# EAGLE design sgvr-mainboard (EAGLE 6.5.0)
CNAME: SGVR Mainboard with Encoder; CREVISION: 1; DESIGNER: Rian Wardana

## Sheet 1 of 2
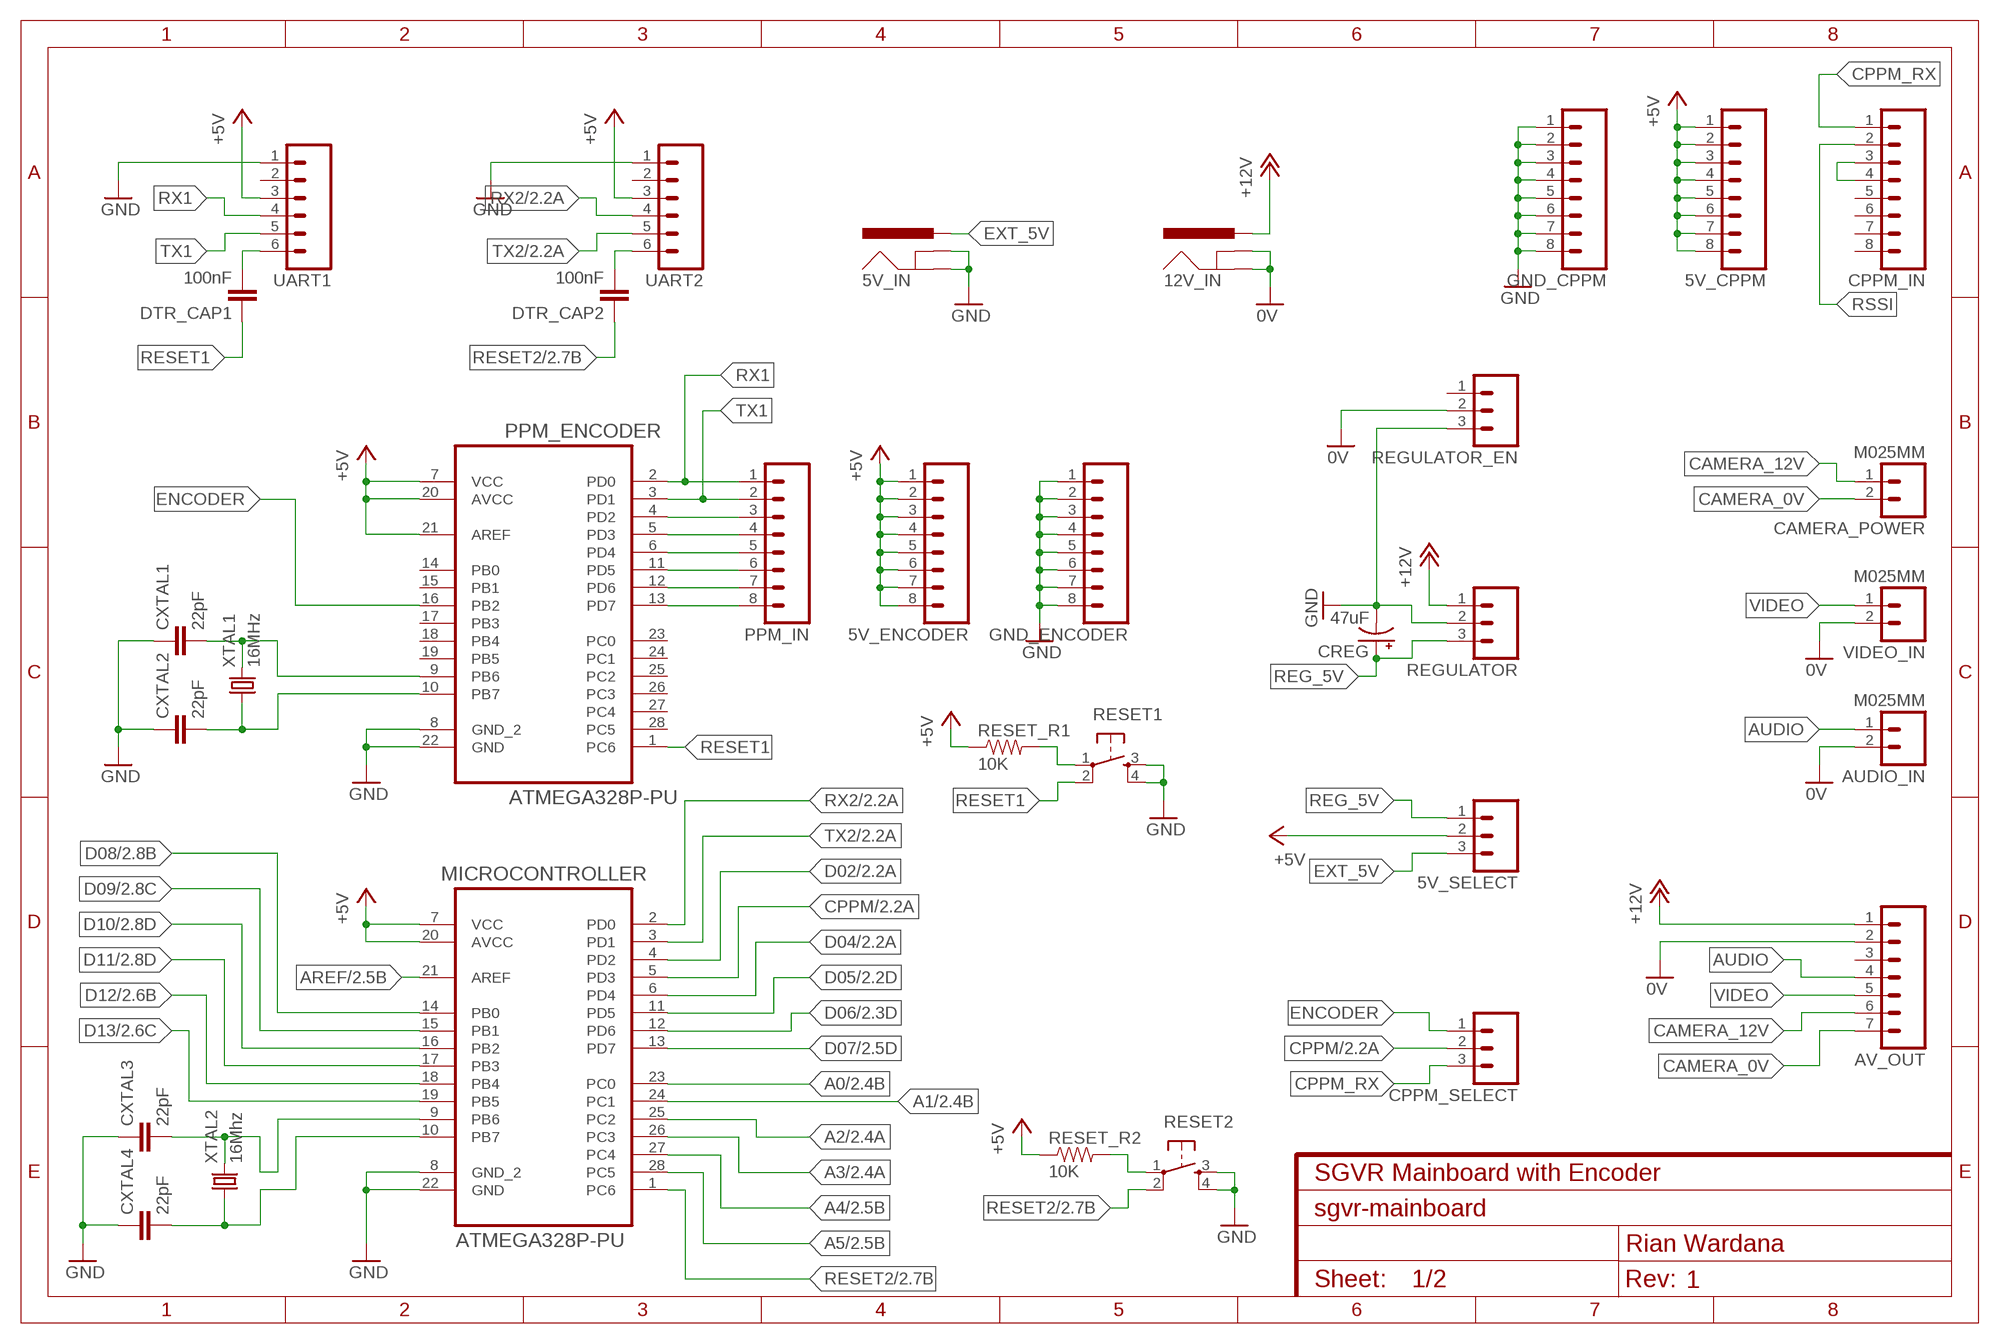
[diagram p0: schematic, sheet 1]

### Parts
5V_CPPM  M08LOCK  [1X08_LOCK]
5V_ENCODER  M08LOCK  [1X08_LOCK]
5V_IN  POWER_JACKPTH_LOCK  [POWER_JACK_PTH_LOCK]
5V_SELECT  M03LOCK_LONGPADS  [1X03_LOCK_LONGPADS]
12V_IN  POWER_JACKPTH_LOCK  [POWER_JACK_PTH_LOCK]
AUDIO_IN  M025MM  [SCREWTERMINAL-5MM-2]
AV_OUT  M07LOCK_LONGPADS  [1X07_LOCK_LONGPADS]
CAMERA_POWER  M025MM  [SCREWTERMINAL-5MM-2]
CPPM_IN  M08LOCK  [1X08_LOCK]
CPPM_SELECT  M03LOCK_LONGPADS  [1X03_LOCK_LONGPADS]
CREG  47uF  CAP_POLPTH1  [CPOL-RADIAL-100UF-25V]
CXTAL1  22pF  CAPPTH  [CAP-PTH-SMALL]
CXTAL2  22pF  CAPPTH  [CAP-PTH-SMALL]
CXTAL3  22pF  CAPPTH  [CAP-PTH-SMALL]
CXTAL4  22pF  CAPPTH  [CAP-PTH-SMALL]
DTR_CAP1  100nF  CAPPTH  [CAP-PTH-SMALL]
DTR_CAP2  100nF  CAPPTH  [CAP-PTH-SMALL]
GND_CPPM  M08LOCK  [1X08_LOCK]
GND_ENCODER  M08LOCK  [1X08_LOCK]
MICROCONTROLLER  ATMEGA328P-PU  [DIP254P762X457-28]
PPM_ENCODER  ATMEGA328P-PU  [DIP254P762X457-28]
PPM_IN  M08LOCK  [1X08_LOCK]
REGULATOR  M03LOCK_LONGPADS  [1X03_LOCK_LONGPADS]
REGULATOR_EN  M03LOCK_LONGPADS  [1X03_LOCK_LONGPADS]
RESET1  TAC_SWITCHPTH  [TACTILE-PTH]
RESET2  TAC_SWITCHPTH  [TACTILE-PTH]
RESET_R1  10K  RESISTORAXIAL-0.3  [AXIAL-0.3]
RESET_R2  10K  RESISTORAXIAL-0.3  [AXIAL-0.3]
UART1  M06LOCK_LONGPADS  [1X06_LOCK_LONGPADS]
UART2  M06LOCK_LONGPADS  [1X06_LOCK_LONGPADS]
VIDEO_IN  M025MM  [SCREWTERMINAL-5MM-2]
XTAL1  16MHz  CRYSTALHC49UV  [HC49U-V]
XTAL2  16Mhz  CRYSTALHC49UV  [HC49U-V]

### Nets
+5V: 5V_CPPM.1 5V_CPPM.2 5V_CPPM.3 5V_CPPM.4 5V_CPPM.5 5V_CPPM.6 5V_CPPM.7 5V_CPPM.8 5V_ENCODER.1 5V_ENCODER.2 5V_ENCODER.3 5V_ENCODER.4 5V_ENCODER.5 5V_ENCODER.6 5V_ENCODER.7 5V_ENCODER.8 5V_SELECT.2 MICROCONTROLLER.7(VCC) MICROCONTROLLER.20(AVCC) PPM_ENCODER.7(VCC) PPM_ENCODER.20(AVCC) PPM_ENCODER.21(AREF) RESET_R1.P$1 RESET_R2.P$1 UART1.3 UART2.3 ; also sheet 2
+12V: 12V_IN.PWR AV_OUT.1 REGULATOR.1
A0: MICROCONTROLLER.23(PC0) ; also sheet 2
A1: MICROCONTROLLER.24(PC1) ; also sheet 2
A2: MICROCONTROLLER.25(PC2) ; also sheet 2
A3: MICROCONTROLLER.26(PC3) ; also sheet 2
A4: MICROCONTROLLER.27(PC4) ; also sheet 2
A5: MICROCONTROLLER.28(PC5) ; also sheet 2
AREF: MICROCONTROLLER.21(AREF) ; also sheet 2
AUDIO: AUDIO_IN.1 AV_OUT.4
CAMERA_0V: AV_OUT.7 CAMERA_POWER.2
CAMERA_12V: AV_OUT.6 CAMERA_POWER.1
CPPM: CPPM_SELECT.2 MICROCONTROLLER.5(PD3) ; also sheet 2
CPPM_RX: CPPM_IN.1 CPPM_SELECT.3
D02: MICROCONTROLLER.4(PD2) ; also sheet 2
D04: MICROCONTROLLER.6(PD4) ; also sheet 2
D05: MICROCONTROLLER.11(PD5) ; also sheet 2
D06: MICROCONTROLLER.12(PD6) ; also sheet 2
D07: MICROCONTROLLER.13(PD7) ; also sheet 2
D08: MICROCONTROLLER.14(PB0) ; also sheet 2
D09: MICROCONTROLLER.15(PB1) ; also sheet 2
D10: MICROCONTROLLER.16(PB2) ; also sheet 2
D11: MICROCONTROLLER.17(PB3) ; also sheet 2
D12: MICROCONTROLLER.18(PB4) ; also sheet 2
D13: MICROCONTROLLER.19(PB5) ; also sheet 2
DTR: DTR_CAP1.2 UART1.6
DTR1: DTR_CAP2.2 UART2.6
ENCODER: CPPM_SELECT.1 PPM_ENCODER.16(PB2)
EXT_5V: 5V_IN.PWR 5V_SELECT.3
GND: 5V_IN.GND 5V_IN.GNDBREAK CREG.2(-) CXTAL1.1 CXTAL2.1 CXTAL3.1 CXTAL4.1 GND_CPPM.1 GND_CPPM.2 GND_CPPM.3 GND_CPPM.4 GND_CPPM.5 GND_CPPM.6 GND_CPPM.7 GND_CPPM.8 GND_ENCODER.1 GND_ENCODER.2 GND_ENCODER.3 GND_ENCODER.4 GND_ENCODER.5 GND_ENCODER.6 GND_ENCODER.7 GND_ENCODER.8 MICROCONTROLLER.8(GND_2) MICROCONTROLLER.22(GND) PPM_ENCODER.8(GND_2) PPM_ENCODER.22(GND) REGULATOR.2 REGULATOR_EN.3 RESET1.3 RESET1.4 RESET2.3 RESET2.4 UART1.1 UART2.1 ; also sheet 2
GROUND12: 12V_IN.GND 12V_IN.GNDBREAK AUDIO_IN.2 AV_OUT.2 REGULATOR_EN.2 VIDEO_IN.2 ; supply symbol labelled 0V
N$1: CXTAL1.2 PPM_ENCODER.9(PB6) XTAL1.2
N$2: CXTAL2.2 PPM_ENCODER.10(PB7) XTAL1.1
N$3: CXTAL3.2 MICROCONTROLLER.9(PB6) XTAL2.2
N$4: CXTAL4.2 MICROCONTROLLER.10(PB7) XTAL2.1
N$7: PPM_ENCODER.4(PD2) PPM_IN.3
N$8: PPM_ENCODER.5(PD3) PPM_IN.4
N$9: PPM_ENCODER.6(PD4) PPM_IN.5
N$10: PPM_ENCODER.11(PD5) PPM_IN.6
N$11: PPM_ENCODER.12(PD6) PPM_IN.7
N$12: PPM_ENCODER.13(PD7) PPM_IN.8
N$13: RESET2.1 RESET_R2.P$2
N$14: CPPM_IN.3 CPPM_IN.4
N$15: RESET1.1 RESET_R1.P$2
REG_5V: 5V_SELECT.1 CREG.1(+) REGULATOR.3
RESET1: DTR_CAP1.1 PPM_ENCODER.1(PC6) RESET1.2
RESET2: DTR_CAP2.1 MICROCONTROLLER.1(PC6) RESET2.2 ; also sheet 2
RSSI: CPPM_IN.2
RX1: PPM_ENCODER.2(PD0) PPM_IN.1 UART1.4
RX2: MICROCONTROLLER.2(PD0) UART2.4 ; also sheet 2
TX1: PPM_ENCODER.3(PD1) PPM_IN.2 UART1.5
TX2: MICROCONTROLLER.3(PD1) UART2.5 ; also sheet 2
VIDEO: AV_OUT.5 VIDEO_IN.1
Unconnected: AV_OUT.3 CPPM_IN.5 CPPM_IN.6 CPPM_IN.7 CPPM_IN.8 PPM_ENCODER.14(PB0) PPM_ENCODER.15(PB1) PPM_ENCODER.17(PB3) PPM_ENCODER.18(PB4) PPM_ENCODER.19(PB5) PPM_ENCODER.23(PC0) PPM_ENCODER.24(PC1) PPM_ENCODER.25(PC2) PPM_ENCODER.26(PC3) PPM_ENCODER.27(PC4) PPM_ENCODER.28(PC5) REGULATOR_EN.1 UART1.2 UART2.2

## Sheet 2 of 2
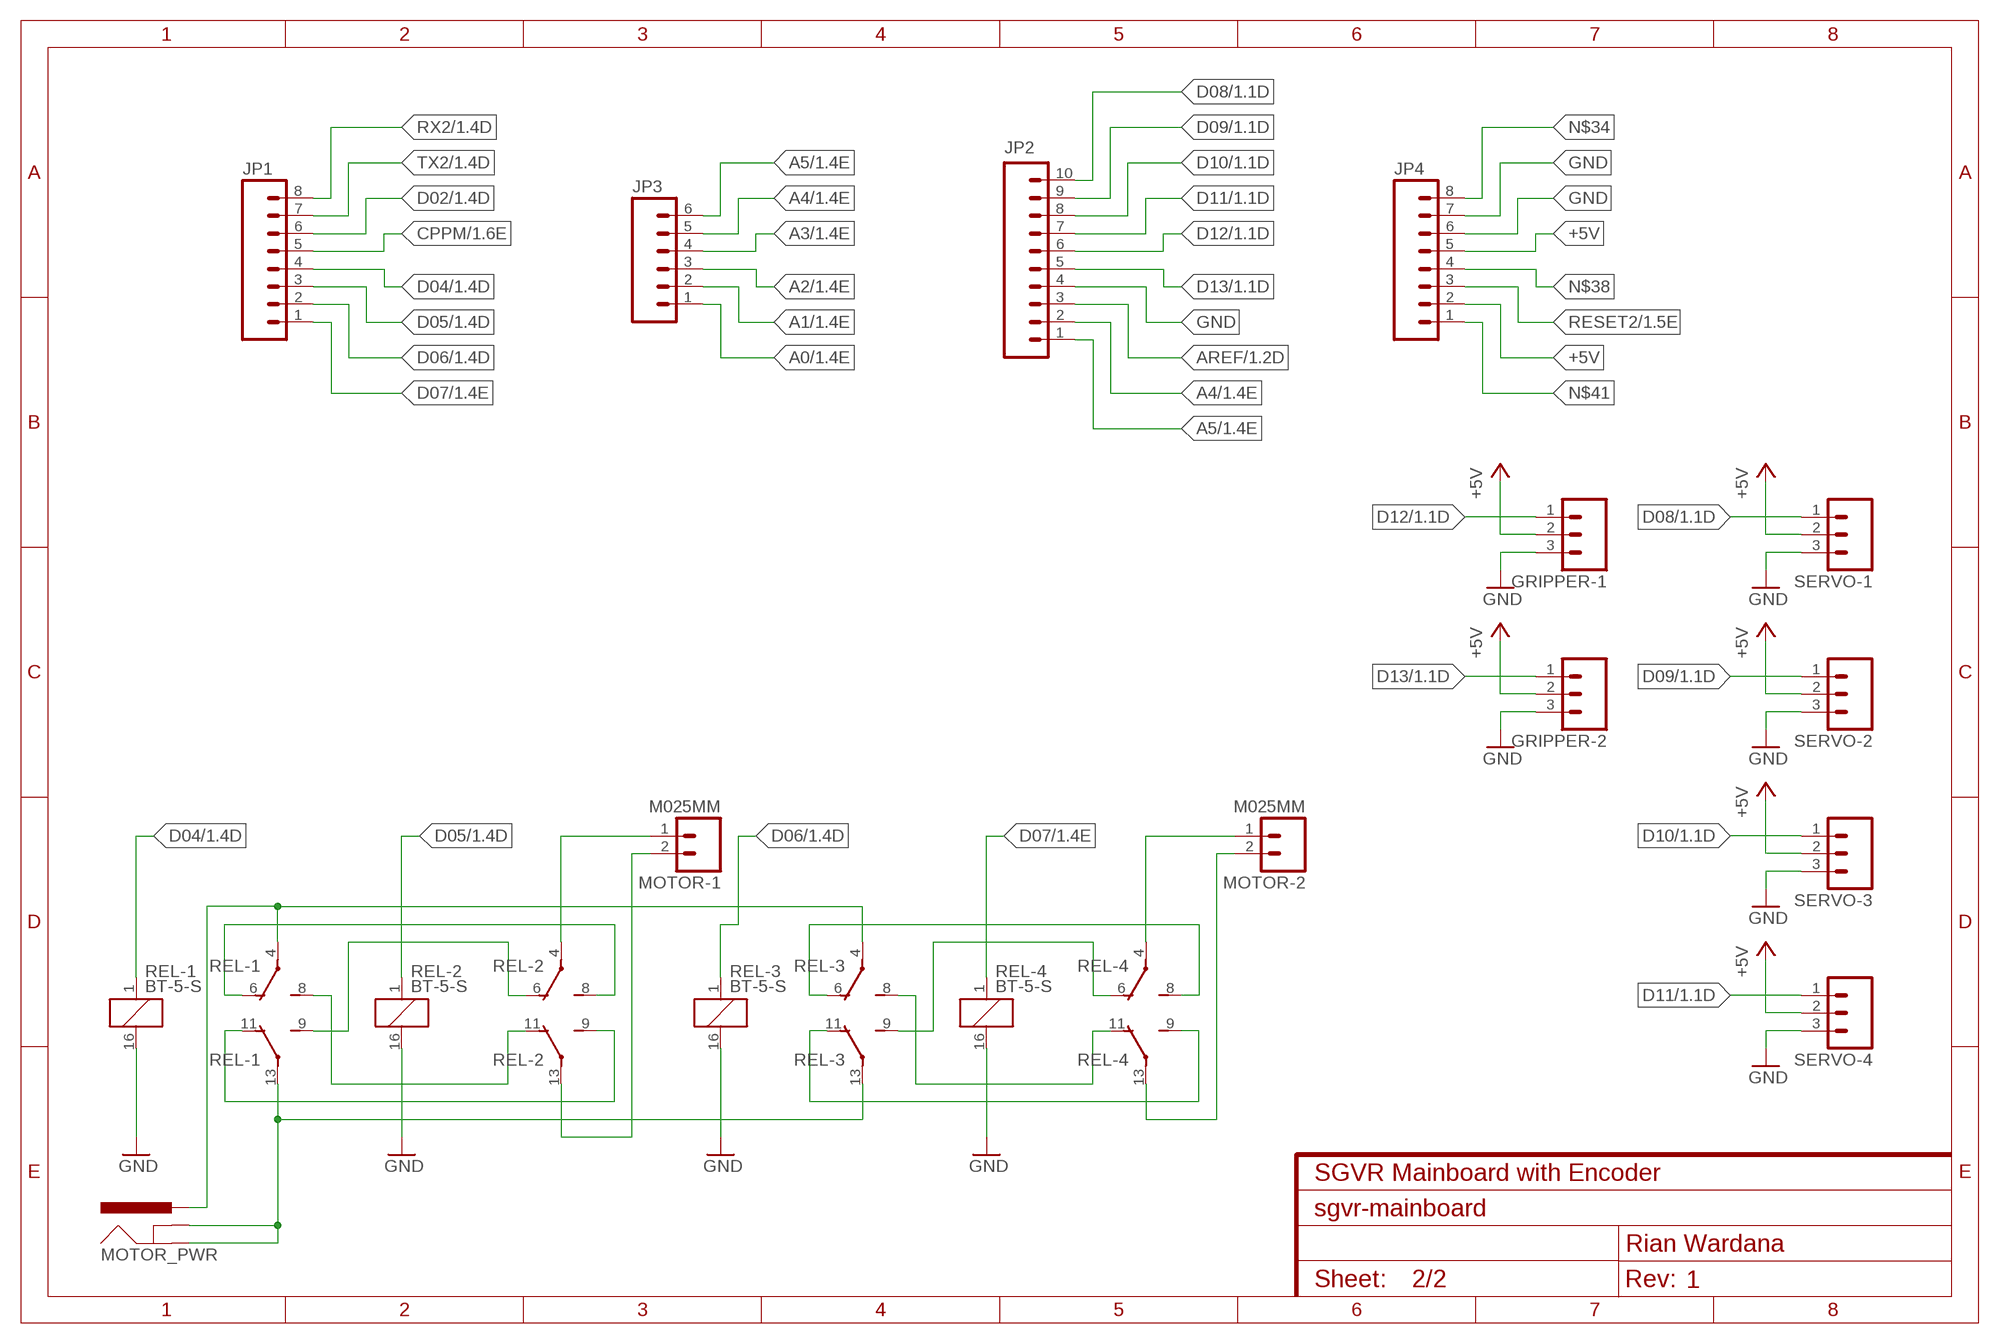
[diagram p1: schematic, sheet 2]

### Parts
GRIPPER-1  M03LOCK_LONGPADS  [1X03_LOCK_LONGPADS]
GRIPPER-2  M03LOCK_LONGPADS  [1X03_LOCK_LONGPADS]
JP1  M08LOCK_LONGPADS  [1X08_LOCK_LONGPADS]
JP2  M10LOCK_LONGPADS  [1X10_LOCK_LONGPADS]
JP3  M06LOCK_LONGPADS  [1X06_LOCK_LONGPADS]
JP4  M08LOCK_LONGPADS  [1X08_LOCK_LONGPADS]
MOTOR-1  M025MM  [SCREWTERMINAL-5MM-2]
MOTOR-2  M025MM  [SCREWTERMINAL-5MM-2]
MOTOR_PWR  POWER_JACKPTH_LOCK  [POWER_JACK_PTH_LOCK]
REL-1  BT-5-S  [BT-XX-S]
REL-2  BT-5-S  [BT-XX-S]
REL-3  BT-5-S  [BT-XX-S]
REL-4  BT-5-S  [BT-XX-S]
SERVO-1  M03LOCK_LONGPADS  [1X03_LOCK_LONGPADS]
SERVO-2  M03LOCK_LONGPADS  [1X03_LOCK_LONGPADS]
SERVO-3  M03LOCK_LONGPADS  [1X03_LOCK_LONGPADS]
SERVO-4  M03LOCK_LONGPADS  [1X03_LOCK_LONGPADS]

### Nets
+5V: GRIPPER-1.2 GRIPPER-2.2 JP4.2 JP4.5 SERVO-1.2 SERVO-2.2 SERVO-3.2 SERVO-4.2 ; also sheet 1
A0: JP3.1 ; also sheet 1
A1: JP3.2 ; also sheet 1
A2: JP3.3 ; also sheet 1
A3: JP3.4 ; also sheet 1
A4: JP2.2 JP3.5 ; also sheet 1
A5: JP2.1 JP3.6 ; also sheet 1
AREF: JP2.3 ; also sheet 1
CPPM: JP1.5 ; also sheet 1
D02: JP1.6 ; also sheet 1
D04: JP1.4 REL-1.1 ; also sheet 1
D05: JP1.3 REL-2.1 ; also sheet 1
D06: JP1.2 REL-3.1 ; also sheet 1
D07: JP1.1 REL-4.1 ; also sheet 1
D08: JP2.10 SERVO-1.1 ; also sheet 1
D09: JP2.9 SERVO-2.1 ; also sheet 1
D10: JP2.8 SERVO-3.1 ; also sheet 1
D11: JP2.7 SERVO-4.1 ; also sheet 1
D12: GRIPPER-1.1 JP2.6 ; also sheet 1
D13: GRIPPER-2.1 JP2.5 ; also sheet 1
GND: GRIPPER-1.3 GRIPPER-2.3 JP2.4 JP4.6 JP4.7 REL-1.16 REL-2.16 REL-3.16 REL-4.16 SERVO-1.3 SERVO-2.3 SERVO-3.3 SERVO-4.3 ; also sheet 1
N$5: REL-3.11(-2:O) REL-4.9(-2:S)
N$6: REL-3.6(-1:O) REL-4.8(-1:S)
N$18: MOTOR-2.1 REL-4.4(-1:P)
N$19: MOTOR-2.2 REL-4.13(-2:P)
N$20: REL-3.9(-2:S) REL-4.6(-1:O)
N$21: REL-3.8(-1:S) REL-4.11(-2:O)
N$22: REL-1.11(-2:O) REL-2.9(-2:S)
N$23: REL-1.6(-1:O) REL-2.8(-1:S)
N$24: MOTOR_PWR.PWR REL-1.4(-1:P) REL-3.4(-1:P)
N$25: MOTOR_PWR.GND MOTOR_PWR.GNDBREAK REL-1.13(-2:P) REL-3.13(-2:P)
N$26: MOTOR-1.1 REL-2.4(-1:P)
N$27: MOTOR-1.2 REL-2.13(-2:P)
N$28: REL-1.9(-2:S) REL-2.6(-1:O)
N$29: REL-1.8(-1:S) REL-2.11(-2:O)
N$34: JP4.8
N$38: JP4.4
N$41: JP4.1
RESET2: JP4.3 ; also sheet 1
RX2: JP1.8 ; also sheet 1
TX2: JP1.7 ; also sheet 1

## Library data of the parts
5V_CPPM 5V_ENCODER CPPM_IN GND_CPPM GND_ENCODER JP1 JP4 PPM_IN = SparkFun-Connectors:M08: Header 8 Standard 8-pin 0.1" header. Use with straight break away headers (SKU : PRT-00116), right angle break away headers (PRT-00553), swiss pins (PRT-00743), machine pins (PRT-00117), and female headers (PRT-00115).
5V_IN 12V_IN MOTOR_PWR = SparkFun-Connectors:POWER_JACK: Power Jack This is the standard 5.5mm barrel jack for power. The PTH is the most common, proven, reliable, footprint. The Slot footprint only works if the mill layer is transmitted to the PCB fab house so be warned. Mating wall wart : TOL-00298 (and others); PROD_ID: PRT-00119
5V_SELECT CPPM_SELECT GRIPPER-1 GRIPPER-2 REGULATOR REGULATOR_EN SERVO-1-SERVO-4 = SparkFun-Connectors:M03: Header 3 Standard 3-pin 0.1" header. Use with straight break away headers (SKU : PRT-00116), right angle break away headers (PRT-00553), swiss pins (PRT-00743), machine pins (PRT-00117), and female headers (PRT-00115). Molex polarized connector foot print use with SKU : PRT-08232 with associated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
AUDIO_IN CAMERA_POWER MOTOR-1 MOTOR-2 VIDEO_IN = SparkFun-Connectors:M02: Standard 2-pin 0.1" header. Use with
AV_OUT = SparkFun-Connectors:M07: Header 7 Standard 7-pin 0.1" header. Use with straight break away headers (SKU : PRT-00116), right angle break away headers (PRT-00553), swiss pins (PRT-00743), machine pins (PRT-00117), and female headers (PRT-00115). NOTES ON THE VARIANTS LOCK and LOCK_LONGPADS... This footprint was designed to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
CREG = SparkFun-Passives:CAP_POL: Capacitor Polarized
CXTAL1 CXTAL2 = SparkFun-Passives:CAP: Capacitor
CXTAL3 CXTAL4 DTR_CAP1 DTR_CAP2 = SparkFun-Capacitors:CAP: Capacitor
JP2 = SparkFun-Connectors:M10: Header 10 Standard 10-pin 0.1" header. Use with straight break away headers (SKU : PRT-00116), right angle break away headers (PRT-00553), swiss pins (PRT-00743), machine pins (PRT-00117), and female headers (PRT-00115).
JP3 UART1 UART2 = SparkFun-Connectors:M06: Header 6 Standard 6-pin 0.1" header. Use with straight break away headers (SKU : PRT-00116), right angle break away headers (PRT-00553), swiss pins (PRT-00743), machine pins (PRT-00117), and female headers (PRT-00115). Molex polarized connector foot print use with SKU : PRT-08094 with associated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
MICROCONTROLLER PPM_ENCODER = Atmel_By_element14_Batch_1-00:ATMEGA328P-PU: 8-bit Microcontroller with In-System Programmable Flash; MPN: ATMEGA328P-PU; OC_FARNELL: 1715487; OC_NEWARK: 15R0268; PACKAGE: PDIP-28; SUPPLIER: Atmel
REL-1-REL-4 = relay:BT-*-S: KLEIN RELAIS WASCHDICHT 2 Wechsler Distriibutor: Conrad Electronic, Bestell Nr.: 505226-13 - 24V 505226-13 - 5V 505170-13 - 12V 505170-13 - 48V Bestar Electric Ltd. Source: http://www2.produktinfo.conrad.com/datenblaetter/500000-524999/505226-da-01-en-Kleinrelais_waschdicht_24V.pdf; OC_FARNELL: unknown; OC_NEWARK: unknown
RESET1 RESET2 = SparkFun-Electromechanical:TAC_SWITCH: Momentary Switch Button commonly used for reset or general input. Spark Fun Electronics SKU : COM-00097 SMT- SWCH-08247
RESET_R1 RESET_R2 = SparkFun-Resistors:RESISTOR: Resistor
XTAL1 XTAL2 = SparkFun-FreqCtrl:CRYSTAL: Various standard crystals. Proven footprints. Spark Fun Electronics SKU : COM-00534

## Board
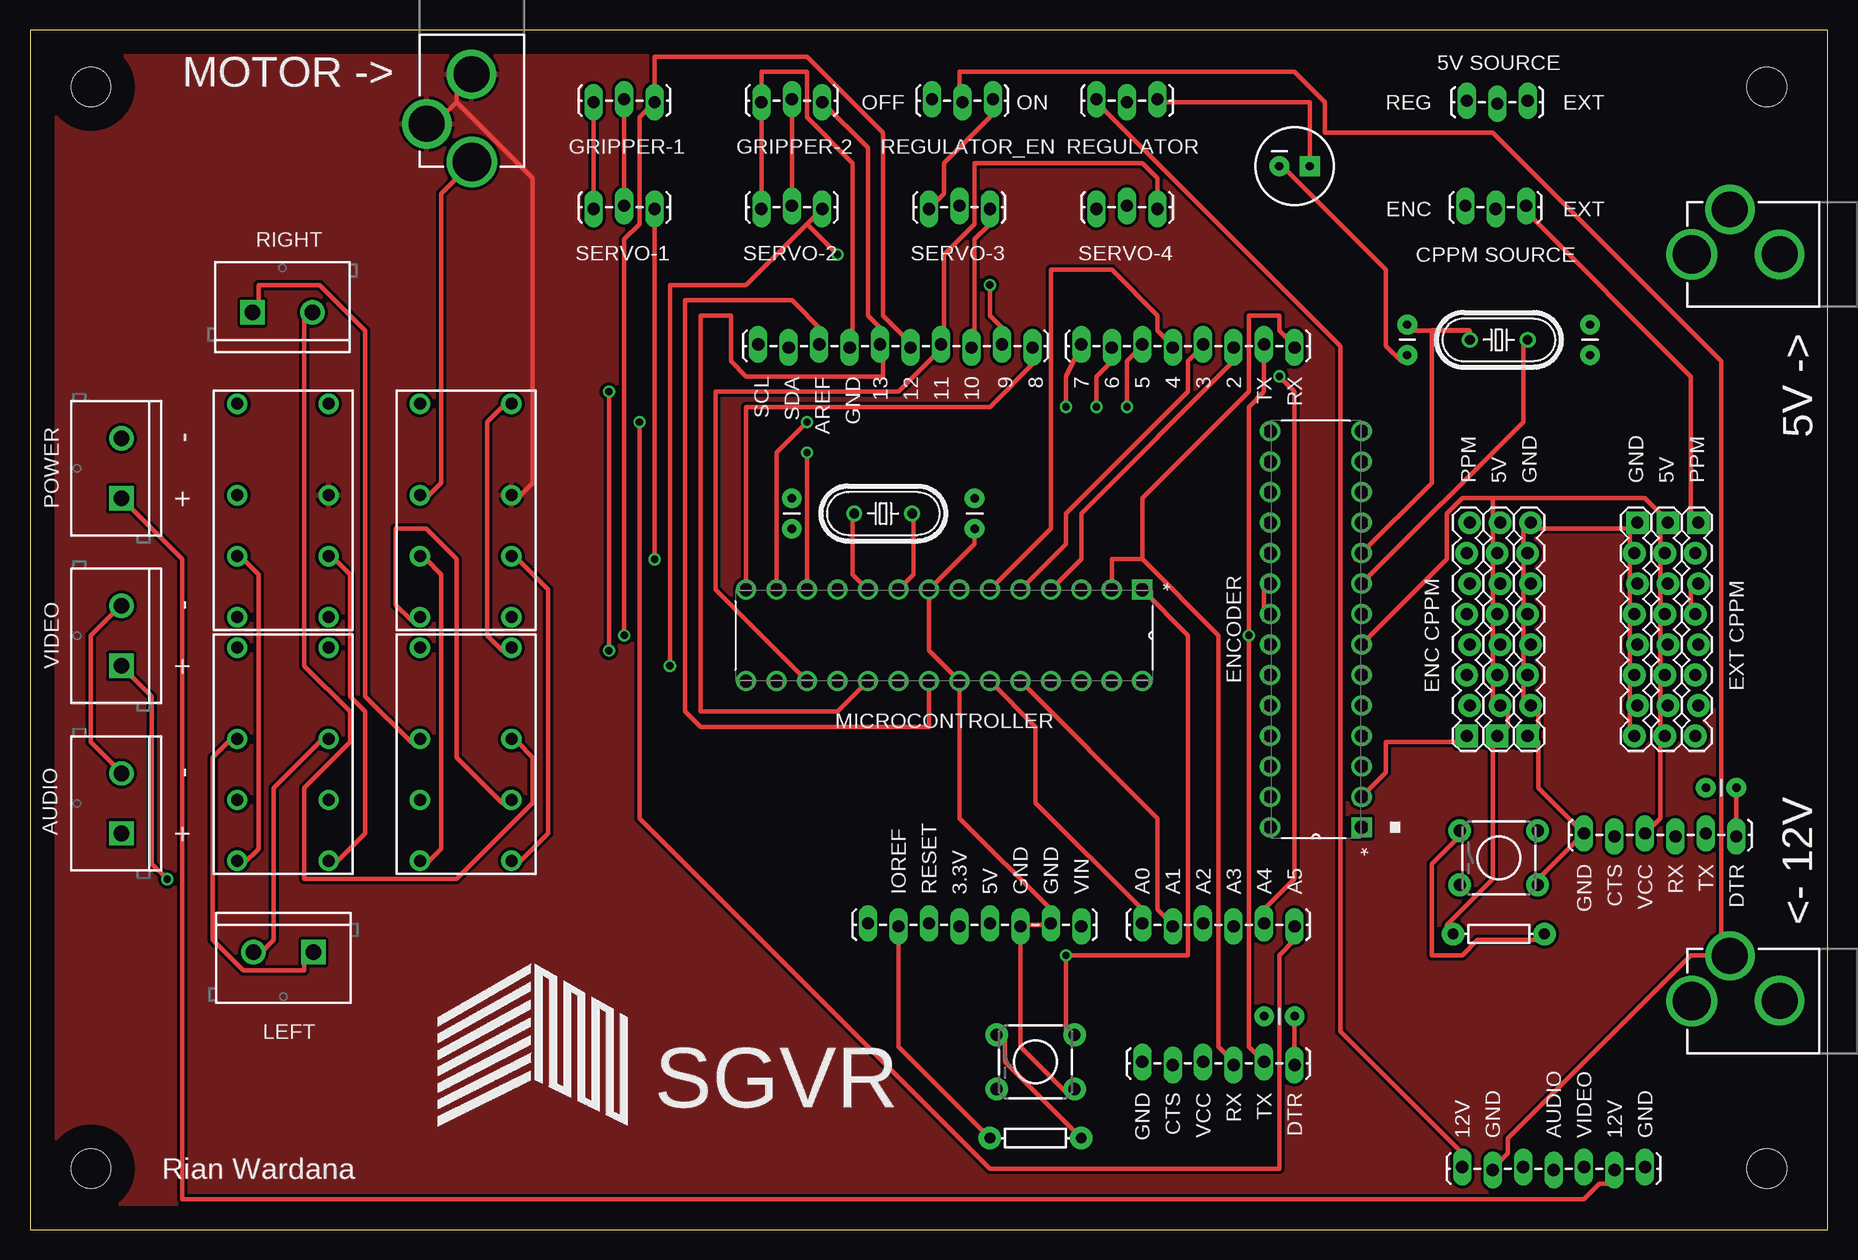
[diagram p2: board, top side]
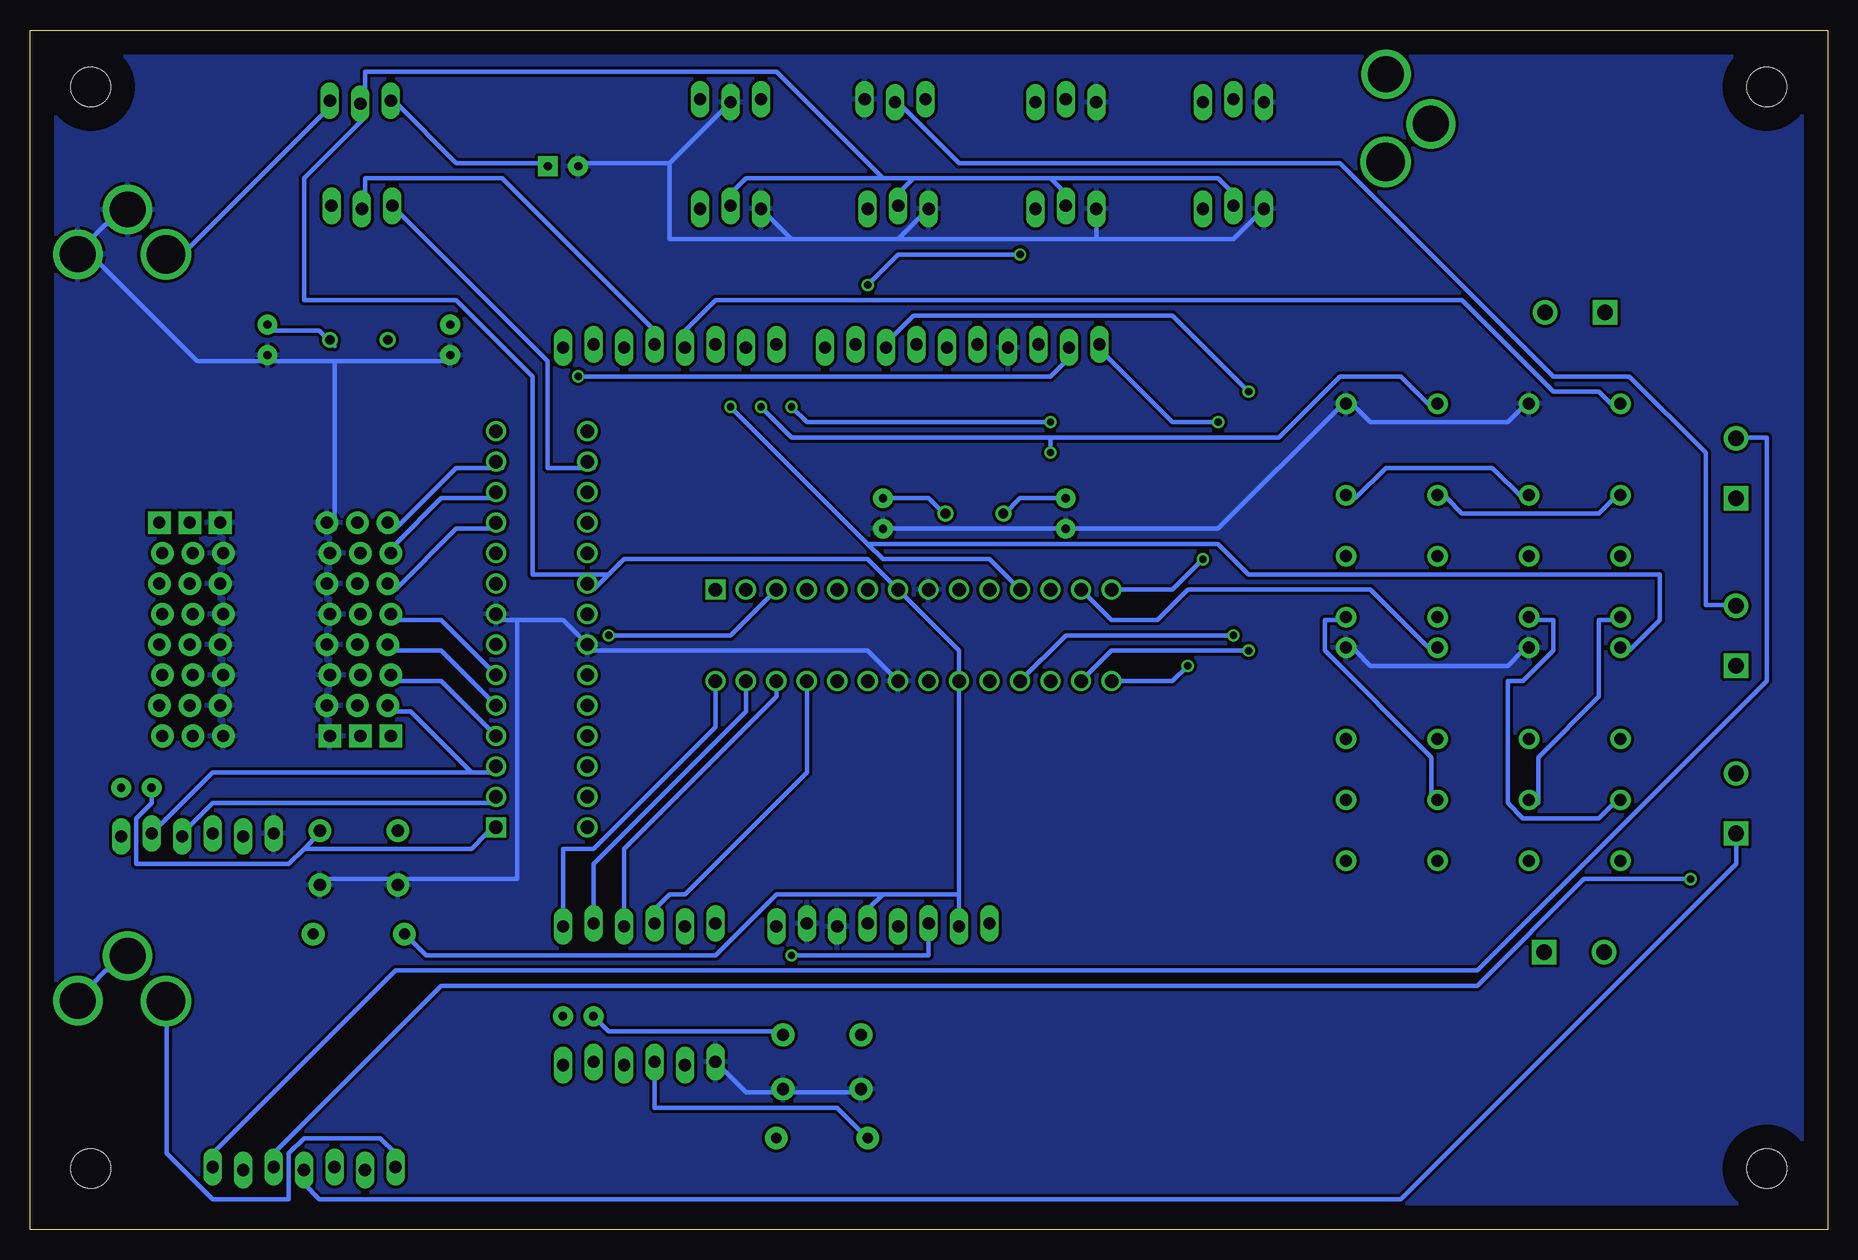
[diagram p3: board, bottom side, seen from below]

Size 149.84 x 100 mm. Coordinates in mm from the lower left corner, seen from the top.
Outline: 0,0 149.84,0 149.84,100 0,100 0,0
Copper layers (1*16): Top 0.035mm / dielectric 1.5mm / Bottom 0.035mm
Design rules "Mazmood *": minimum track width 15mil, minimum drill 24mil, track to track 10mil, track to pad 10mil, pad to pad 10mil, via to via 10mil, smd to smd 10mil, copper to edge 2mm, drill to drill 10mil, minimum pad ring 10mil, minimum via ring 8mil, stop-mask expansion 4mil, vias tented up to drill 0mil, thermal gap 10mil

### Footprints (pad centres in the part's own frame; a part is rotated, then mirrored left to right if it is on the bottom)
1X08_LOCK = drill 1.016 pad 1.88 square: 1 0,0.127 | drill 1.016 pad 1.88: 2 2.54,-0.127; 3 5.08,0.127; 4 7.62,-0.127; 5 10.16,0.127; 6 12.7,-0.127; 7 15.24,0.127; 8 17.78,-0.127
POWER_JACK_PTH_LOCK = drill 2.997 pad 4.115: GND 0.025,6.557; GNDBREAK 3.762,10.7 | drill 3.2 pad 4.115: PWR 0,13.878
1X03_LOCK_LONGPADS = drill 1.016 long: 1 0,0; 2 2.54,-0.254; 3 5.08,0
SCREWTERMINAL-5MM-2 = drill 1.3 pad 2.032 square: 1 0,0 | drill 1.3 pad 2.032: 2 5,0
1X07_LOCK_LONGPADS = drill 1.016 long: 1 0,0.127; 2 2.54,-0.127; 3 5.08,0.127; 4 7.62,-0.127; 5 10.16,0.127; 6 12.7,-0.127; 7 15.24,0.127
CPOL-RADIAL-100UF-25V = drill 0.7 pad 1.651 square: 1 1.27,0 | drill 0.7 pad 1.651: 2 -1.27,0
CAP-PTH-SMALL = drill 0.7 pad 1.651: 1 0,0; 2 2.54,0
1X08_LOCK_LONGPADS = drill 1.016 long: 1 0,0.127; 2 2.54,-0.127; 3 5.08,0.127; 4 7.62,-0.127; 5 10.16,0.127; 6 12.7,-0.127; 7 15.24,0.127; 8 17.78,-0.127
1X10_LOCK_LONGPADS = drill 1.016 long: 1 0,0.127; 2 2.54,-0.127; 3 5.08,0.127; 4 7.62,-0.127; 5 10.16,0.127; 6 12.7,-0.127; 7 15.24,0.127; 8 17.78,-0.127; 9 20.32,0.127; 10 22.86,-0.127
1X06_LOCK_LONGPADS = drill 1.016 long: 1 0,0; 2 2.54,-0.254; 3 5.08,0; 4 7.62,-0.254; 5 10.16,0; 6 12.7,-0.254
DIP254P762X457-28 = drill 1.118 square: 1 -7.62,33.02 | drill 1.118: 2 -7.62,30.48; 3 -7.62,27.94; 4 -7.62,25.4; 5 -7.62,22.86; 6 -7.62,20.32; 7 -7.62,17.78; 8 -7.62,15.24; 9 -7.62,12.7; 10 -7.62,10.16; 11 -7.62,7.62; 12 -7.62,5.08; 13 -7.62,2.54; 14 -7.62,0; 15 0,0; 16 0,2.54; 17 0,5.08; 18 0,7.62; 19 0,10.16; 20 0,12.7; 21 0,15.24; 22 0,17.78; 23 0,20.32; 24 0,22.86; 25 0,25.4; 26 0,27.94; 27 0,30.48; 28 0,33.02
BT-XX-S = drill 1 pad 1.7: 1 -8.89,-3.81; 4 -1.27,-3.81; 6 3.81,-3.81; 8 8.89,-3.81; 9 8.89,3.81; 11 3.81,3.81; 13 -1.27,3.81; 16 -8.89,3.81
TACTILE-PTH = drill 1.016 pad 1.88: 1 -3.251,2.261; 2 3.251,2.261; 3 -3.251,-2.261; 4 3.251,-2.261
AXIAL-0.3 = drill 0.9 pad 1.88: P$1 -3.81,0; P$2 3.81,0
STAND-OFF = hole 3.302: 0,0
HC49U-V = drill 0.813: 1 -2.413,0; 2 2.413,0

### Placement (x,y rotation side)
5V_CPPM  136.4,58.93 270 top
5V_ENCODER  122.43,41.15 90 top
5V_IN  152.4,81.28 90 top
5V_SELECT  119.76,94.11 0 top
12V_IN  152.4,19.05 90 top
AUDIO_IN  7.62,33.02 90 top
AV_OUT  119.38,5.08 0 top
CAMERA_POWER  7.62,60.96 90 top
CPPM_IN  138.94,58.93 270 top
CPPM_SELECT  119.63,85.34 0 top
CREG  105.41,88.65 0 top
CXTAL1  130.05,72.9 90 top
CXTAL2  114.81,72.9 90 top
CXTAL3  78.74,58.42 90 top
CXTAL4  63.5,58.42 90 top
DTR_CAP1  139.7,36.83 0 top
DTR_CAP2  102.87,17.78 0 top
GND_CPPM  133.86,58.93 270 top
GND_ENCODER  124.97,41.15 90 top
GRIPPER-1  52.07,93.98 180 top
GRIPPER-2  66.04,93.98 180 top
JP1  87.63,73.66 0 top
JP2  60.71,73.66 0 top
JP3  92.71,25.53 0 top
JP4  69.85,25.4 0 top
MICROCONTROLLER  59.69,45.72 270 top
MOTOR-1  23.62,23.11 180 top
MOTOR-2  18.54,76.45 0 top
MOTOR_PWR  36.83,102.87 180 top
PPM_ENCODER  103.38,66.55 180 top
PPM_IN  119.89,41.15 90 top
REGULATOR  88.9,94.23 0 top
REGULATOR_EN  75.18,94.23 0 top
REL-1  21.08,59.94 270 top
REL-2  21.08,39.62 270 top
REL-3  36.32,59.94 270 top
REL-4  36.32,39.62 270 top
RESET1  122.43,30.99 0 top
RESET2  83.82,13.97 0 top
RESET_R1  122.43,24.64 0 top
RESET_R2  83.82,7.62 0 top
SERVO-1  52.07,85.09 180 top
SERVO-2  66.04,85.09 180 top
SERVO-3  80.01,85.09 180 top
SERVO-4  93.98,85.09 180 top
U$1  [STAND-OFF]  5.08,5.08 0 top
U$2  [STAND-OFF]  5.08,95.25 0 top
U$3  [STAND-OFF]  144.78,5.08 0 top
U$4  [STAND-OFF]  144.78,95.25 0 top
UART1  129.54,33.02 0 top
UART2  92.71,13.97 0 top
VIDEO_IN  7.62,46.99 90 top
XTAL1  122.43,74.17 0 top
XTAL2  71.12,59.69 0 top

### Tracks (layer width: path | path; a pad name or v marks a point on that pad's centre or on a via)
+5V
  Top 0.381: GRIPPER-1.2 SERVO-1.2 | GRIPPER-2.2 SERVO-2.2 | 135.89,53.34 135.89,52.07 5V_CPPM.4 135.89,50.8 135.89,48.26 | 135.89,48.26 135.89,46.99 5V_CPPM.6 135.89,45.72 135.89,43.18 | UART1.3 135.89,34.29 135.89,40.64 5V_CPPM.8 135.89,41.91 135.89,43.18 | 135.89,43.18 5V_CPPM.7 | 135.89,48.26 5V_CPPM.5 | 135.89,53.34 135.89,55.88 5V_CPPM.2 135.89,57.15 135.89,58.42 5V_CPPM.1 135.89,59.69 134.62,60.96 121.92,60.96 | 135.89,53.34 5V_CPPM.3 | 121.92,60.96 119.38,60.96 118.11,59.69 118.11,55.88 PPM_ENCODER.7 110.49,48.26 | 121.92,58.42 121.92,60.96 | 121.92,58.42 121.92,57.15 5V_ENCODER.7 121.92,55.88 121.92,53.34 | 121.92,58.42 5V_ENCODER.8 | 121.92,53.34 121.92,52.07 5V_ENCODER.5 121.92,50.8 121.92,48.26 | 121.92,48.26 121.92,46.99 5V_ENCODER.3 121.92,45.72 121.92,43.18 5V_ENCODER.2 123.19,43.18 123.19,41.91 5V_ENCODER.1 121.92,40.64 121.92,29.21 118.11,25.4 RESET_R1.P$1 | 121.92,48.26 5V_ENCODER.4 | 121.92,53.34 5V_ENCODER.6 | PPM_ENCODER.21 102.87,50.8 102.87,53.34 PPM_ENCODER.20 | RESET_R2.P$1 72.39,15.24 JP4.2
  Bottom 0.381: 76.2,87.63 77.47,86.36 SERVO-3.2 | 64.77,87.63 76.2,87.63 | 64.77,87.63 63.5,86.36 SERVO-2.2 | 76.2,87.63 78.74,87.63 | 78.74,87.63 90.17,87.63 91.44,86.36 SERVO-4.2 | 78.74,87.63 87.63,96.52 121.92,96.52 121.92,93.98 5V_SELECT.2 121.92,92.71 127,87.63 127,77.47 114.3,77.47 107.95,71.12 107.95,54.61 101.6,54.61 | 64.77,87.63 50.8,87.63 49.53,86.36 SERVO-1.2 | UART2.3 97.79,10.16 82.55,10.16 RESET_R2.P$1 | 72.39,27.94 MICROCONTROLLER.20 72.39,48.26 MICROCONTROLLER.7 80.01,55.88 100.33,55.88 101.6,54.61 | 72.39,27.94 JP4.2 | 78.74,27.94 80.01,26.67 JP4.5 | 72.39,27.94 78.74,27.94 | 101.6,54.61 102.87,53.34 PPM_ENCODER.20 | RESET_R1.P$1 116.84,22.86 92.71,22.86 87.63,27.94 78.74,27.94
+12V
  Top 0.381: REGULATOR.1 88.9,93.98 109.22,73.66 109.22,16.51 119.38,6.35 AV_OUT.1
  Bottom 0.381: AV_OUT.1 119.38,6.35 120.65,7.62 127,7.62 128.27,6.35 128.27,2.54 134.62,2.54 138.43,6.35 138.43,19.05 12V_IN.PWR
A0
  Top 0.381: MICROCONTROLLER.23 83.82,41.91 83.82,35.56 92.71,26.67 JP3.1
A1
  Top 0.381: MICROCONTROLLER.24 93.98,34.29 93.98,26.67 95.25,25.4 JP3.2
A2
  Bottom 0.381: MICROCONTROLLER.25 85.09,38.1 95.25,27.94 96.52,27.94 97.79,26.67 JP3.3
A3
  Bottom 0.381: JP3.4 100.33,31.75 87.63,44.45 MICROCONTROLLER.26
A4  (via drill 0.61)
  Top 0.381: v104.14,71.12 105.41,69.85 105.41,29.21 102.87,26.67 JP3.5
  Bottom 0.381: JP3.5 102.87,30.48 90.17,43.18 MICROCONTROLLER.27 | v104.14,71.12 64.77,71.12 63.5,72.39 JP2.2
A5  (via drill 0.61)
  Top 0.381: v50.8,67.31 50.8,34.29 80.01,5.08 104.14,5.08 104.14,22.86 105.41,24.13 JP3.6
  Bottom 0.381: JP3.6 105.41,31.75 102.87,31.75 92.71,41.91 MICROCONTROLLER.28 | v50.8,67.31 54.61,67.31 60.96,73.66 JP2.1
AREF
  Top 0.381: MICROCONTROLLER.21 74.93,41.91 55.88,41.91 54.61,43.18 54.61,77.47 63.5,77.47 66.04,74.93 JP2.3
AUDIO
  Bottom 0.381: AUDIO_IN.1 7.62,30.48 35.56,2.54 125.73,2.54 127,3.81 AV_OUT.4
CAMERA_0V
  Bottom 0.381: AV_OUT.7 134.62,6.35 119.38,21.59 29.21,21.59 5.08,45.72 5.08,66.04 7.62,66.04 CAMERA_POWER.2
CAMERA_12V
  Top 0.381: CAMERA_POWER.1 12.7,55.88 12.7,2.54 129.54,2.54 130.81,3.81 132.08,3.81 AV_OUT.6
CPPM
  Top 0.381: MICROCONTROLLER.5 86.36,57.15 86.36,59.69 96.52,69.85 96.52,72.39 97.79,73.66 JP1.5
  Bottom 0.381: CPPM_SELECT.2 121.92,85.09 121.92,87.63 110.49,87.63 97.79,74.93 JP1.5
CPPM_RX
  Top 0.381: CPPM_SELECT.3 124.46,85.09 138.43,71.12 138.43,59.69 CPPM_IN.1
D02
  Top 0.381: MICROCONTROLLER.4 87.63,55.88 87.63,59.69 100.33,72.39 JP1.6
D04
  Top 0.381: MICROCONTROLLER.6 85.09,58.42 85.09,80.01 90.17,80.01 93.98,76.2 93.98,74.93 95.25,73.66 JP1.4
  Bottom 0.381: JP1.4 95.25,74.93 92.71,77.47 30.48,77.47 22.86,69.85 19.05,69.85 17.78,68.58 REL-1.1
D05  (via drill 0.61)
  Top 0.381: v91.44,68.58 91.44,72.39 92.71,73.66 JP1.3
  Bottom 0.381: 80.01,57.15 78.74,55.88 69.85,55.88 MICROCONTROLLER.11 | 80.01,57.15 v91.44,68.58 | 80.01,57.15 50.8,57.15 48.26,54.61 13.97,54.61 13.97,50.8 16.51,48.26 REL-2.1
D06  (via drill 0.61)
  Top 0.381: v88.9,68.58 88.9,71.12 90.17,72.39 JP1.2 | v64.77,64.77 MICROCONTROLLER.12
  Bottom 0.381: v88.9,68.58 86.36,66.04 64.77,66.04 | 64.77,66.04 45.72,66.04 40.64,71.12 35.56,71.12 33.02,68.58 REL-3.1 | 64.77,66.04 v64.77,64.77
D07  (via drill 0.61)
  Top 0.381: JP1.1 86.36,71.12 v86.36,68.58 | v64.77,67.31 62.23,64.77 MICROCONTROLLER.13
  Bottom 0.381: v86.36,68.58 85.09,67.31 v64.77,67.31 | MICROCONTROLLER.13 59.69,50.8 55.88,50.8 53.34,53.34 38.1,53.34 33.02,48.26 REL-4.1
D08  (via drill 0.61)
  Top 0.381: v52.07,55.88 SERVO-1.1 | MICROCONTROLLER.14 59.69,68.58 80.01,68.58 83.82,72.39 JP2.10
  Bottom 0.381: v52.07,55.88 54.61,53.34 MICROCONTROLLER.14
D09  (via drill 0.61)
  Top 0.381: 64.77,83.82 59.69,78.74 53.34,78.74 v53.34,46.99 | 64.77,83.82 SERVO-2.1 | v80.01,78.74 80.01,76.2 81.28,74.93 JP2.9 | 64.77,83.82 v67.31,81.28
  Bottom 0.381: v53.34,46.99 54.61,45.72 MICROCONTROLLER.15 | v80.01,78.74 77.47,81.28 v67.31,81.28
D10  (via drill 0.61)
  Top 0.381: SERVO-3.1 80.01,83.82 78.74,82.55 78.74,73.66 JP2.8 | v48.26,69.85 v48.26,48.26
  Bottom 0.381: MICROCONTROLLER.16 59.69,48.26 v48.26,48.26 | v48.26,69.85 54.61,76.2 76.2,76.2 78.74,73.66 JP2.8
D11
  Top 0.381: MICROCONTROLLER.17 57.15,53.34 57.15,69.85 72.39,69.85 76.2,73.66 JP2.7 76.2,74.93 76.2,81.28 78.74,83.82 78.74,88.9 92.71,88.9 93.98,87.63 SERVO-4.1
D12  (via drill 0.61)
  Top 0.381: JP2.6 73.66,73.66 71.12,76.2 71.12,91.44 64.77,97.79 52.07,97.79 GRIPPER-1.1 50.8,92.71 50.8,83.82 49.53,82.55 v49.53,49.53
  Bottom 0.381: MICROCONTROLLER.18 63.5,49.53 v49.53,49.53
D13
  Top 0.381: GRIPPER-2.1 69.85,90.17 69.85,76.2 71.12,74.93 JP2.5 71.12,73.66 71.12,71.12 59.69,71.12 58.42,72.39 58.42,76.2 55.88,76.2 55.88,43.18 67.31,43.18 MICROCONTROLLER.19
DTR
  Top 0.381: DTR_CAP1.2 UART1.6
DTR1
  Top 0.381: DTR_CAP2.2 UART2.6
ENCODER
  Bottom 0.381: CPPM_SELECT.1 106.68,72.39 106.68,63.5 102.87,63.5 PPM_ENCODER.16
EXT_5V
  Bottom 0.381: 5V_IN.PWR 137.16,81.28 124.46,93.98 5V_SELECT.3
GND
  Top 0.381: REL-4.16 39.37,48.26 38.1,49.53 38.1,67.31 39.37,68.58 REL-3.16 | CXTAL3.1 78.74,57.15 MICROCONTROLLER.8 74.93,48.26 MICROCONTROLLER.22 77.47,34.29 85.09,26.67 JP4.7 85.09,25.4 82.55,25.4 JP4.6 82.55,15.24 86.36,11.43 RESET2.4 | SERVO-2.3 GRIPPER-2.3 60.96,96.52 64.77,96.52 64.77,92.71 68.58,88.9 68.58,73.66 JP2.4 | GRIPPER-1.3 SERVO-1.3 | SERVO-3.3 76.2,86.36 76.2,88.9 80.01,92.71 80.01,93.98 REGULATOR_EN.3 | RESET1.4 125.73,29.21 UART1.1 125.73,36.83 125.73,40.64 GND_ENCODER.1 125.73,41.91 125.73,43.18 GND_ENCODER.2 124.46,43.18 124.46,45.72 GND_ENCODER.3 124.46,46.99 124.46,48.26 | 133.35,58.42 133.35,57.15 GND_CPPM.2 133.35,55.88 133.35,53.34 | 133.35,53.34 133.35,52.07 GND_CPPM.4 133.35,50.8 133.35,48.26 | 133.35,43.18 133.35,41.91 GND_CPPM.8 | 133.35,48.26 133.35,46.99 GND_CPPM.6 133.35,45.72 133.35,43.18 | 133.35,43.18 GND_CPPM.7 | 133.35,48.26 GND_CPPM.5 | 133.35,53.34 GND_CPPM.3 | 124.46,53.34 124.46,52.07 GND_ENCODER.5 124.46,50.8 124.46,48.26 | 124.46,48.26 GND_ENCODER.4 | 124.46,53.34 124.46,55.88 GND_ENCODER.7 124.46,57.15 124.46,58.42 GND_ENCODER.8 125.73,58.42 133.35,58.42 | 124.46,53.34 GND_ENCODER.6 | 133.35,58.42 GND_CPPM.1 | CREG.2 104.14,88.9 113.03,80.01 113.03,73.66 114.3,72.39 CXTAL2.1
  Bottom 0.381: REL-2.16 25.4,48.26 26.67,46.99 38.1,46.99 39.37,48.26 REL-4.16 | REL-1.16 25.4,68.58 26.67,67.31 38.1,67.31 39.37,68.58 REL-3.16 40.64,68.58 50.8,58.42 CXTAL4.1 CXTAL3.1 | UART2.1 90.17,11.43 87.63,11.43 RESET2.4 86.36,11.43 81.28,11.43 RESET2.3 | 96.52,88.9 REGULATOR.2 | 96.52,88.9 104.14,88.9 CREG.2 | 86.36,82.55 SERVO-4.3 | 77.47,82.55 86.36,82.55 | SERVO-3.3 77.47,82.55 | SERVO-1.3 49.53,82.55 60.96,82.55 | 77.47,82.55 60.96,82.55 | 96.52,88.9 96.52,82.55 86.36,82.55 | 60.96,82.55 SERVO-2.3 | 109.22,50.8 110.49,50.8 PPM_ENCODER.8 | 109.22,50.8 105.41,50.8 PPM_ENCODER.22 102.87,48.26 80.01,48.26 MICROCONTROLLER.22 | 119.38,29.21 125.73,29.21 RESET1.4 | 109.22,50.8 109.22,29.21 119.38,29.21 | 119.38,29.21 RESET1.3 | 5V_IN.GNDBREAK 142.24,83.82 143.51,83.82 144.78,82.55 5V_IN.GND 144.78,81.28 135.89,72.39 129.54,72.39 | 129.54,72.39 124.46,72.39 | 124.46,72.39 114.3,72.39 CXTAL2.1 | 124.46,72.39 124.46,58.42 GND_ENCODER.8 | 129.54,72.39 CXTAL1.1
  pour Bottom: -1.27,-1.27 153.67,-1.27 153.67,104.14 -1.27,104.14
GROUND12
  Top 0.381: 140.97,22.86 138.43,22.86 123.19,7.62 123.19,6.35 121.92,5.08 AV_OUT.2 | AUDIO_IN.2 7.62,38.1 5.08,40.64 5.08,49.53 7.62,52.07 VIDEO_IN.2 | 140.97,22.86 140.97,72.39 121.92,91.44 107.95,91.44 107.95,93.98 105.41,96.52 77.47,96.52 77.47,93.98 REGULATOR_EN.2 | 140.97,22.86 12V_IN.GNDBREAK
  Bottom 0.381: 12V_IN.GND 144.78,20.32 143.51,21.59 142.24,21.59 12V_IN.GNDBREAK | REGULATOR_EN.2 77.47,93.98 72.39,88.9 40.64,88.9 22.86,71.12 16.51,71.12 10.16,64.77 10.16,52.07 7.62,52.07 VIDEO_IN.2
N$1
  Top 0.381: 110.49,53.34 PPM_ENCODER.9 124.46,67.31 124.46,73.66 XTAL1.2
  Bottom 0.381: XTAL1.2 124.46,73.66 125.73,74.93 129.54,74.93 CXTAL1.2
N$2
  Top 0.381: CXTAL2.2 114.3,74.93 116.84,74.93 116.84,62.23 PPM_ENCODER.10 110.49,55.88
  Top 0.406: XTAL1.1 120.02,74.93 116.84,74.93
N$3
  Top 0.381: MICROCONTROLLER.9 73.66,54.61 73.66,59.69 XTAL2.2
  Bottom 0.381: CXTAL3.2 74.93,60.96 73.66,59.69 XTAL2.2
N$4
  Top 0.381: MICROCONTROLLER.10 68.58,54.61 68.58,59.69 XTAL2.1
  Bottom 0.381: CXTAL4.2 67.31,60.96 68.58,59.69 XTAL2.1
N$5
  Top 0.381: REL-4.9 40.64,30.48 43.18,33.02 43.18,53.34 40.64,55.88 REL-3.11
N$6
  Top 0.381: REL-4.8 33.02,30.48 34.29,31.75 34.29,54.61 33.02,55.88 REL-3.6
N$7
  Bottom 0.381: 110.49,40.64 PPM_ENCODER.4 115.57,45.72 119.38,45.72 PPM_IN.3
N$8
  Bottom 0.381: 110.49,43.18 PPM_ENCODER.5 115.57,48.26 119.38,48.26 PPM_IN.4
N$9
  Bottom 0.381: 110.49,45.72 PPM_ENCODER.6 115.57,50.8 119.38,50.8 PPM_IN.5
N$10
  Bottom 0.381: PPM_ENCODER.11 110.49,58.42 114.3,58.42 119.38,53.34 PPM_IN.6
N$11
  Bottom 0.381: PPM_ENCODER.12 110.49,60.96 115.57,60.96 119.38,57.15 PPM_IN.7
N$12
  Bottom 0.381: PPM_ENCODER.13 110.49,63.5 114.3,63.5 119.38,58.42 PPM_IN.8
N$13
  Top 0.381: RESET_R2.P$2 81.28,13.97 81.28,16.51 RESET2.1
N$14
  Top 0.381: CPPM_IN.4 138.43,52.07 138.43,53.34 CPPM_IN.3
N$15
  Top 0.381: RESET_R1.P$2 125.73,24.13 120.65,24.13 119.38,22.86 116.84,22.86 116.84,30.48 119.38,33.02 RESET1.1
N$18
  Top 0.381: REL-4.4 31.75,40.64 27.94,44.45 27.94,74.93 24.13,78.74 19.05,78.74 19.05,76.2 MOTOR-2.1
N$19
  Top 0.381: REL-4.13 40.64,40.64 41.91,39.37 41.91,35.56 35.56,29.21 22.86,29.21 22.86,36.83 26.67,40.64 26.67,43.18 22.86,46.99 22.86,76.2 MOTOR-2.2
N$20
  Bottom 0.381: REL-4.6 33.02,35.56 33.02,39.37 41.91,48.26 41.91,50.8 40.64,50.8 REL-3.9
N$21
  Top 0.381: REL-4.11 39.37,35.56 35.56,39.37 35.56,55.88 33.02,58.42 30.48,58.42 30.48,52.07 31.75,50.8 REL-3.8
N$22
  Top 0.381: REL-2.9 25.4,30.48 27.94,33.02 27.94,43.18 26.67,44.45 26.67,54.61 25.4,55.88 REL-1.11
N$23
  Top 0.381: REL-2.8 17.78,30.48 19.05,31.75 19.05,54.61 17.78,55.88 REL-1.6
N$24
  Top 0.381: MOTOR_PWR.PWR 36.83,88.9 34.29,86.36 34.29,62.23 33.02,60.96 REL-3.4
  Bottom 0.381: REL-1.4 17.78,60.96 19.05,59.69 30.48,59.69 31.75,60.96 REL-3.4
N$25
  Top 0.381: 35.56,93.98 34.29,92.71 MOTOR_PWR.GNDBREAK | 35.56,93.98 35.56,95.25 MOTOR_PWR.GND | 35.56,93.98 41.91,87.63 41.91,62.23 40.64,60.96 REL-3.13
  Bottom 0.381: REL-1.13 25.4,60.96 27.94,63.5 36.83,63.5 39.37,60.96 REL-3.13
  pour Top: -2.54,-2.54 154.94,-2.54 154.94,105.41 -2.54,105.41
N$26
  Top 0.381: REL-2.4 16.51,40.64 15.24,39.37 15.24,24.13 17.78,21.59 22.86,21.59 22.86,22.86 MOTOR-1.1
N$27
  Top 0.381: REL-2.13 24.13,40.64 20.32,36.83 20.32,24.13 19.05,22.86 MOTOR-1.2
N$28
  Bottom 0.381: REL-2.6 17.78,35.56 19.05,34.29 25.4,34.29 26.67,35.56 26.67,45.72 25.4,45.72 22.86,48.26 22.86,50.8 24.13,50.8 REL-1.9
N$29
  Bottom 0.381: REL-2.11 24.13,35.56 24.13,39.37 19.05,44.45 19.05,50.8 17.78,50.8 REL-1.8
REG_5V
  Top 0.381: CREG.1 106.68,93.98 93.98,93.98 REGULATOR.3
  Bottom 0.381: 5V_SELECT.1 119.38,93.98 114.3,88.9 106.68,88.9 CREG.1
RESET1
  Bottom 0.381: DTR_CAP1.1 139.7,35.56 140.97,34.29 140.97,30.48 128.27,30.48 127,31.75 | 127,31.75 125.73,33.02 RESET1.2 | 127,31.75 113.03,31.75 111.76,33.02 PPM_ENCODER.1
RESET2  (via drill 0.61)
  Top 0.381: RESET2.2 86.36,16.51 v86.36,22.86 96.52,22.86 96.52,49.53 MICROCONTROLLER.1
  Bottom 0.381: JP4.3 74.93,22.86 v86.36,22.86 | DTR_CAP2.1 101.6,16.51 87.63,16.51 RESET2.2
RX1
  Top 0.381: PPM_IN.1 119.38,40.64 113.03,40.64 113.03,38.1 PPM_ENCODER.2 110.49,35.56
  Bottom 0.381: UART1.4 137.16,33.02 134.62,35.56 110.49,35.56 PPM_ENCODER.2
RX2
  Top 0.381: 92.71,55.88 99.06,49.53 99.06,15.24 100.33,13.97 UART2.4 | 92.71,55.88 90.17,55.88 MICROCONTROLLER.2 | 92.71,55.88 92.71,60.96 101.6,69.85 101.6,76.2 104.14,76.2 104.14,74.93 105.41,73.66 JP1.8
TX1
  Bottom 0.381: UART1.5 134.62,38.1 113.03,38.1 | 113.03,38.1 110.49,38.1 PPM_ENCODER.3 | 113.03,38.1 118.11,43.18 119.38,43.18 PPM_IN.2
TX2  (via drill 0.61)
  Top 0.381: UART2.5 101.6,15.24 v101.6,49.53 101.6,68.58 102.87,69.85 JP1.7
  Bottom 0.381: MICROCONTROLLER.3 91.44,49.53 v101.6,49.53
VIDEO  (via drill 0.61)
  Top 0.381: v11.43,29.21 10.16,30.48 10.16,44.45 VIDEO_IN.1
  Bottom 0.381: v11.43,29.21 20.32,29.21 29.21,20.32 115.57,20.32 129.54,6.35 AV_OUT.5

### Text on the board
tPlace: MOTOR -> | OFF | ON | RIGHT | 5V -> | POWER | PPM | 5V | GND | GND | 5V | PPM | VIDEO | ENCODER | ENC CPPM | EXT CPPM | MICROCONTROLLER | AUDIO | . | GND | CTS | VCC | RX | TX | DTR | <- 12V | LEFT | SGVR | GND | CTS | VCC | RX | TX | DTR | 12V | GND | AUDIO | VIDEO | 12V | GND | Rian Wardana | C:/Users/Frederick Gum/Documents/DipTrace/Eagle/Projects/logo.bmp
tNames: 5V SOURCE | REG | EXT | ENC | EXT | CPPM SOURCE | SCL | SDA | AREF | GND | 13 | 12 | 11 | 10 | 9 | 8 | 7 | 6 | 5 | 4 | 3 | 2 | TX | RX | - | + | - | + | - | + | IOREF | RESET | 3.3V | 5V | GND | GND | VIN | A0 | A1 | A2 | A3 | A4 | A5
